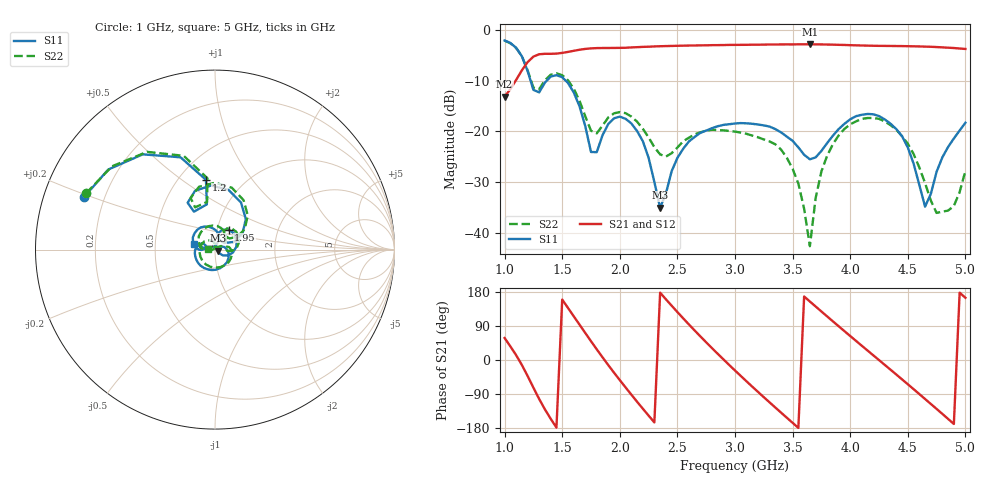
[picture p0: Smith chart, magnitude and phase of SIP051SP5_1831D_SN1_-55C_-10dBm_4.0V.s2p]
# GHz  S  dB  R  50
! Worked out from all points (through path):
!   81 points, 1 GHz to 5 GHz, reference 50 ohm
!   highest |S21| = -2.84 dB at 3.65 GHz (marker M1); lowest = -13.2 dB at 1 GHz (marker M2)
!   lowest |S11| = -35.1 dB at 2.35 GHz (marker M3), VSWR 1.04, Z = 51.7 - j0.541 ohm
!   |S11| at or under -10 dB: 1.225 GHz to 1.367 GHz (141.5 MHz wide, 10.9 % of centre); 1.529 GHz to end of sweep
!   |S22| runs from -42.7 to -2.1 dB; largest |S21 - S12| = 0.0018
!   S11 on the Smith chart (normalised r, x): 1 GHz: 0.12, +0.19; 1.2 GHz: 0.67, +0.62; 1.95 GHz: 1.13, +0.26; 5 GHz: 0.79, +0.05
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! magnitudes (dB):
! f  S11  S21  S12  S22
! 1 GHz  -2.1  -13.2  -13.2  -2.1
! 1.2 GHz  -8.1  -6.4  -6.4  -8.0
! 1.3 GHz  -12.3  -4.8  -4.8  -11.7
! 1.5 GHz  -9.3  -4.5  -4.5  -8.9
! 1.7 GHz  -19.0  -3.8  -3.8  -17.0
! 1.8 GHz  -24.1  -3.6  -3.6  -20.4
! 1.95 GHz  -17.4  -3.6  -3.6  -16.5
! 2.2 GHz  -22.0  -3.4  -3.4  -19.5
! 2.35 GHz  -35.1  -3.2  -3.2  -24.6
! 2.6 GHz  -22.0  -3.1  -3.1  -21.3
! 3 GHz  -18.5  -3.0  -2.9  -20.1
! 3.45 GHz  -21.1  -2.9  -2.9  -25.2
! 3.55 GHz  -23.2  -2.8  -2.8  -30.3
! 3.65 GHz  -25.5  -2.8  -2.8  -42.7
! 3.7 GHz  -25.2  -2.9  -2.9  -33.2
! 3.95 GHz  -18.5  -3.0  -3.0  -19.5
! 4.35 GHz  -18.5  -3.2  -3.2  -18.8
! 4.5 GHz  -23.2  -3.2  -3.2  -22.5
! 4.65 GHz  -34.9  -3.3  -3.3  -30.2
! 4.75 GHz  -28.0  -3.4  -3.4  -36.1
! 4.85 GHz  -23.1  -3.5  -3.5  -35.6
! 5 GHz  -18.3  -3.8  -3.8  -27.8
